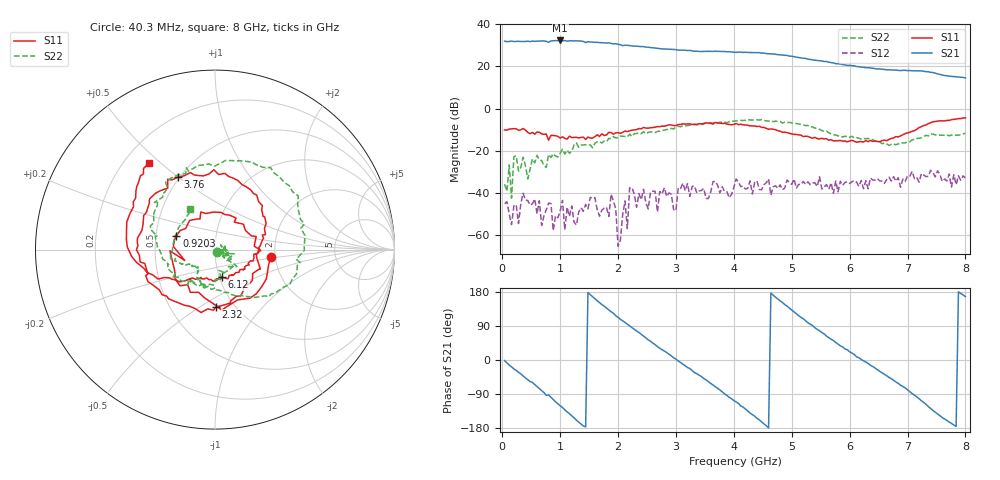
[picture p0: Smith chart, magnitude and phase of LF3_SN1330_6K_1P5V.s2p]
! VC=1.5V I=7.5mA
# HZ S DB R 50.00
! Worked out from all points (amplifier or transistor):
!   200 points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, 40.3 MHz to 8 GHz, reference 50 ohm
!   highest |S21| = 32.3 dB at 1 GHz (marker M1)
!   |S21| within 3 dB of that: start of sweep to 2.455 GHz
!   unconditionally stable (mu >= 1): start of sweep to 3.196 GHz; 3.203 GHz to 3.64 GHz; 4.379 GHz to end of sweep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
!   at 1.36 GHz: K = 2.71, MAG = 32.3 dB, |S12| = -46.9 dB
!   at 4.04 GHz: K = 0.82, MSG = 30.0 dB, |S12| = -33.3 dB
!   at 8 GHz: K = 2.54, MAG = 16.8 dB, |S12| = -32.8 dB
!   S11 on the Smith chart (normalised r, x): 40.3 MHz: 1.90, -0.17; 920.3 MHz: 0.64, +0.10; 2.32 GHz: 0.82, -0.58; 3.76 GHz: 0.49, +0.50; 6.12 GHz: 1.03, -0.33; 8 GHz: 0.30, +0.46
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4.02985e7  -10.06 -7.2  31.99 -1.5  -45.03 -61.1  -35.73 -55.3
4.402835e8  -11.22 -102.4  31.96 -52.0  -43.51 53.9  -33.29 -13.3
7.20273e8  -12.18 -164.8  32.14 -86.1  -50.69 36.1  -27.06 6.6
9.202655e8  -12.82 160.4  32.27 -110.3  -50.78 94.0  -22.42 -11.8
1.000262e9  -13.93 144.1  32.33 -120.7  -48.46 114.3  -21.02 -35.7
1.280252e9  -13.56 80.5  32.15 -158.7  -55.14 70.0  -16.20 -37.7
1.400248e9  -13.51 56.2  31.85 -174.2  -48.64 -15.0  -17.17 -54.4
1.560242e9  -13.95 31.8  31.59 167.0  -42.56 9.5  -18.56 -79.0
1.840231e9  -11.21 -23.2  31.22 132.1  -51.06 -136.1  -14.07 -92.5
2.320213e9  -9.93 -89.0  29.64 76.4  -46.69 -27.0  -11.75 -139.6
2.720198e9  -8.55 -136.0  28.43 31.2  -39.25 -78.9  -10.59 -169.2
3.240178e9  -7.20 171.4  27.63 -22.7  -41.55 168.0  -7.86 142.5
3.760159e9  -6.86 117.1  27.16 -79.2  -39.91 -170.7  -6.42 101.2
4.040148e9  -7.03 90.9  26.68 -110.5  -33.33 -161.5  -5.82 75.1
4.360136e9  -8.23 59.1  26.60 -148.3  -34.86 162.4  -5.38 43.9
4.600128e9  -9.75 34.4  26.02 -179.4  -33.29 112.8  -5.93 19.5
5.000112e9  -11.94 4.9  24.89 132.1  -35.82 93.7  -6.73 -21.2
5.360099e9  -13.99 -22.6  23.13 90.8  -35.23 45.3  -8.68 -45.3
6.12007e9  -15.93 -75.5  19.96 8.5  -34.82 9.4  -13.70 -113.0
6.68005e9  -14.59 -119.5  18.42 -45.9  -32.46 -29.3  -17.39 -134.7
7.240028e9  -8.52 -158.1  17.92 -107.8  -30.74 -78.1  -13.76 -157.3
8e9  -4.35 127.5  14.57 167.3  -32.76 -156.9  -11.60 121.4
